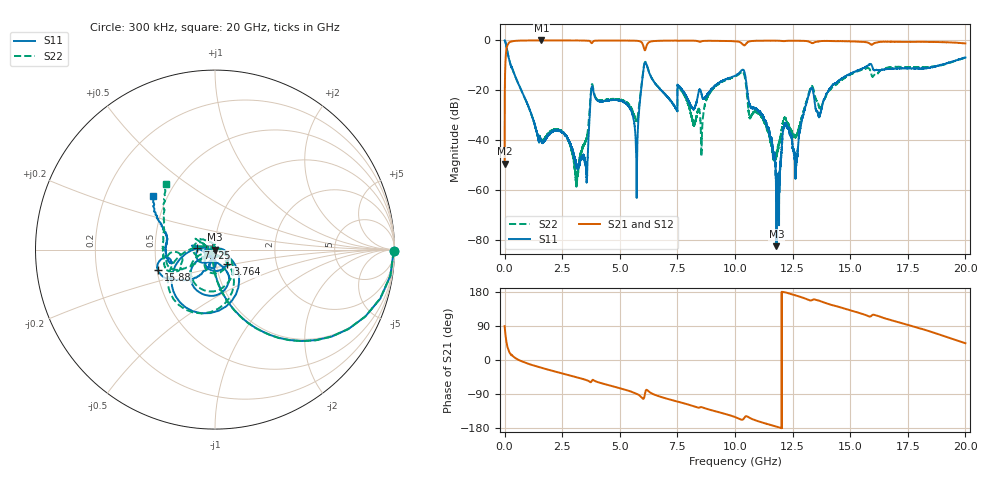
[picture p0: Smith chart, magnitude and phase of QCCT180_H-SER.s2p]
! Created Fri Feb  5 15:32:51 2021
# hz S ma R 50
! 2 Port Network Data from SP1.SP block
! freq  magS11  angS11  magS21  angS21  magS12  angS12  magS22  angS22
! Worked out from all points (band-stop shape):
!   20001 points, 300 kHz to 20 GHz, reference 50 ohm
!   highest |S21| = 0.00 dB at 1.597 GHz (marker M1); lowest = -49.4 dB at 300 kHz (marker M2)
!   |S21| within 3 dB of the highest: 91.13 MHz to 6.046 GHz (5.955 GHz wide, 194 % of centre); 6.133 GHz to end of sweep
!   lowest |S11| = -82.6 dB at 11.8 GHz (marker M3), VSWR 1.00, Z = 50 + j0.00716 ohm
!   |S11| at or under -10 dB: 265.6 MHz to 6.054 GHz (5.789 GHz wide, 183 % of centre); 6.173 GHz to 15.78 GHz (9.602 GHz wide, 87.5 % of centre); 15.94 GHz to 18.87 GHz (2.934 GHz wide, 16.9 % of centre)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
!   |S22| runs from -58.7 to 0.0 dB; largest |S21 - S12| = 0.016
!   S11 on the Smith chart (normalised r, x): 300 kHz: open; 3.764 GHz: 1.13, -0.18; 7.725 GHz: 0.82, +0.02; 15.88 GHz: 0.51, -0.13; 20 GHz: 0.42, +0.31
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300000  0.996 -0.3  0.003375 89.3  0.003326 89.9  0.9957 -0.4
1.723e8  0.4606 -64.7  0.8848 25.3  0.8855 25.2  0.4633 -64.7
1.5973e9  0.00948 -42.5  0.9998 -20.5  0.9986 -20.6  0.01007 178.1
3.3343e9  0.004363 -135.1  0.9978 -49.0  0.9978 -49.0  0.00573 -104.4
3.5603e9  0.001414 139.5  0.9944 -53.3  0.995 -53.3  0.0111 -61.4
3.7643e9  0.1052 -49.0  0.8865 -57.2  0.8878 -57.2  0.1177 -61.5
5.2993e9  0.05299 -178.8  0.9931 -79.7  0.9923 -79.7  0.05681 -154.3
5.7083e9  0.006236 175.6  0.9858 -88.4  0.9852 -88.5  0.02465 -111.8
6.0843e9  0.3549 -94.4  0.6358 -92.0  0.6373 -91.9  0.3632 -101.5
6.6673e9  0.1165 179.2  0.9833 -95.1  0.9839 -95.0  0.117 175.4
7.7253e9  0.09994 174.7  0.9894 -113.4  0.9908 -113.3  0.09121 141.1
8.5583e9  0.08048 -111.0  0.9622 -124.6  0.962 -124.5  0.01038 -5.4
1.00003e10  0.1948 -67.0  0.9642 -150.5  0.9649 -150.4  0.1888 -64.0
1.13843e10  0.01979 -84.2  0.99 -168.6  0.9897 -168.5  0.01715 -85.9
1.18013e10  7.444e-05 106.0  0.9888 -175.8  0.9874 -175.8  0.00467 166.8
1.21573e10  0.02046 131.4  0.9721 178.9  0.9716 178.9  0.02769 130.3
1.26423e10  0.002942 -24.4  0.987 170.2  0.9868 170.2  0.01212 166.2
1.33343e10  0.1113 -157.7  0.8881 157.7  0.89 157.5  0.1227 178.2
1.36583e10  0.02927 -143.3  0.9614 156.4  0.9628 156.4  0.04525 170.1
1.58823e10  0.3369 -160.3  0.8399 114.9  0.8408 115.0  0.242 -176.4
1.66673e10  0.2677 -168.1  0.9429 106.9  0.9319 106.7  0.2867 -155.9
2e10  0.4542 139.3  0.8714 44.2  0.8602 44.0  0.4558 126.7
